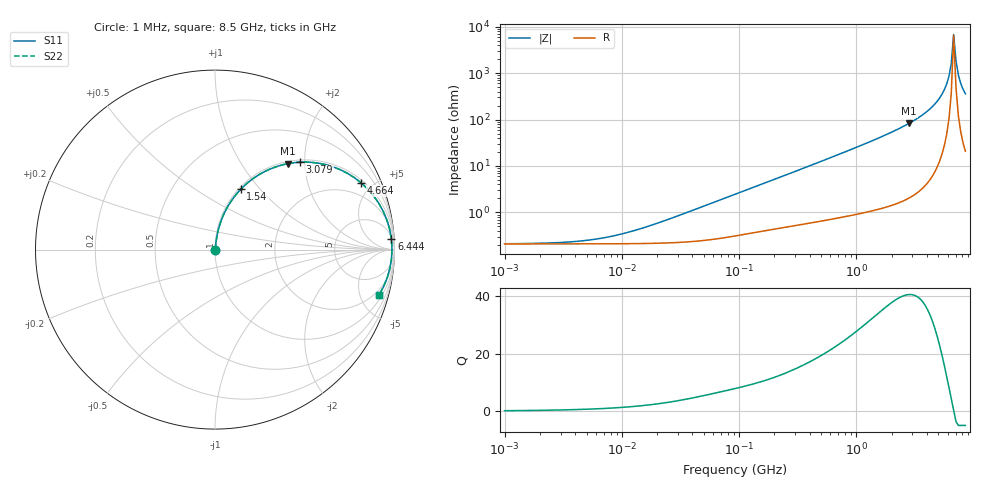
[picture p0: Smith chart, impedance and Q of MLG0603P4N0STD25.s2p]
! S-Parameter Data Generated by TDK Corporation
! Copyright(C) 2025 TDK Corporation.
! All Rights Reserved.
! TDK P/N: MLG0603P4N0STD25 (SMD / SMT Inductor (Coil))
! Property: L=4nH at 500MHz
! Size(LxWxT): 0.6x0.3x0.3mm
! Model Type: s2p (Touchstone File Format Version 1.0)
! Frequency: DC=Yes Start=1MHz Stop=8500MHz 198points Log-sweep
! Model Generated on Feb. 6, 2025
! Terms and conditions regarding TDK Simulation Models:
! 1)This simulation model is being provided solely for informational
!  purposes. Please refer to the specifications of the products in
!  terms of detailed characteristics of such products.
! 2)In no event shall TDK Corporation of any of its subsidiaries be
!  liable for any loss or damage arising, directly or indirectly,
!  from any information contained in this simulation model, including,
!  but not limited to loss or damages arising from any inaccuracies,
!  omissions or errors in connection with such information.
! 3)Any and all copyrights on this simulation model are owned by
!  TDK Corporation.  Duplication or redistribution of this simulation
!  model without prior written permission from TDK Corporation
!  is prohibited.
! 4)This simulation model is subject to any modification or change
!  without any prior notice.
! 5)Neither TDK Corporation nor any of its subsidiaries shall make any
!  warranty, express or implied, including but not limited to the
!  correctness, implied warranties of merchantability and fitness for
!  a particular purpose with respect to this simulation models.
! 6)The use of this simulation model shall be deemed to have consented
!  to the terms and conditions hereof.
! Port Assignments:
!  1 ---@@@--- 2
! Applicable Conditions:
!  Temperature = 25 degC
!  DC Bias Current = 0 A
!  Small Signal Operation
# Hz S MA R 50
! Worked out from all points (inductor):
!   197 points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, 1 MHz to 8.5 GHz, reference 50 ohm
!   read as one part in series: L = 4.31 nH near 25.31 MHz
!   highest Q = 40.6 at 2.807 GHz (marker M1), where L = 4.68 nH
!   self-resonance near 6.748 GHz
!   S11 on the Smith chart (normalised r, x): 1 MHz: 1.00, +0.00; 1.54 GHz: 1.02, +0.80; 3.079 GHz: 1.05, +1.89; 4.664 GHz: 1.15, +4.31; 6.444 GHz: 8, +31; 8.5 GHz: 1.42, -7.13
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1000000  0.002113 7.4  0.9979 -0.0  0.9979 -0.0  0.002113 7.4
4587603  0.002441 30.6  0.9979 -0.1  0.9979 -0.1  0.002441 30.6
9601846  0.003355 50.8  0.9979 -0.1  0.9979 -0.1  0.003355 50.8
2.10461e7  0.006103 68.8  0.9978 -0.3  0.9978 -0.3  0.006103 68.8
9.219544e7  0.0245 81.3  0.9966 -1.4  0.9966 -1.4  0.0245 81.3
4.229561e8  0.1055 80.7  0.9885 -6.0  0.9885 -6.0  0.1055 80.7
9.270694e8  0.2256 74.8  0.9658 -13.0  0.9658 -13.0  0.2256 74.8
1.540426e9  0.3666 66.8  0.9197 -21.5  0.9197 -21.5  0.3666 66.8
1.940355e9  0.4545 61.4  0.8787 -27.0  0.8787 -27.0  0.4545 61.4
2.80715e9  0.6295 49.6  0.7616 -39.0  0.7616 -39.0  0.6295 49.6
3.07866e9  0.6788 45.9  0.7178 -42.7  0.7178 -42.7  0.6788 45.9
3.877948e9  0.8042 34.9  0.5729 -53.5  0.5729 -53.5  0.8042 34.9
4.664383e9  0.8954 24.5  0.4152 -63.5  0.4152 -63.5  0.8954 24.5
5.357206e9  0.9483 15.8  0.2728 -71.3  0.2728 -71.3  0.9483 15.8
5.87536e9  0.972 9.7  0.1688 -75.6  0.1688 -75.6  0.972 9.7
6.152938e9  0.9797 6.6  0.115 -76.6  0.115 -76.6  0.9797 6.6
6.44363e9  0.9844 3.4  0.06093 -73.5  0.06093 -73.5  0.9844 3.4
6.748056e9  0.986 0.2  0.01453 -15.8  0.01453 -15.8  0.986 0.2
7.066863e9  0.9845 -2.9  0.05324 71.7  0.05324 71.7  0.9845 -2.9
7.400733e9  0.98 -6.1  0.1073 76.2  0.1073 76.2  0.98 -6.1
7.750377e9  0.9724 -9.2  0.1612 75.5  0.1612 75.5  0.9724 -9.2
8.5e9  0.9488 -15.4  0.2656 71.3  0.2656 71.3  0.9488 -15.4
